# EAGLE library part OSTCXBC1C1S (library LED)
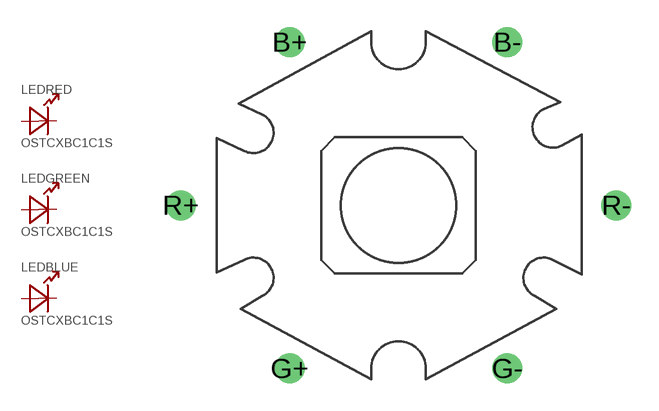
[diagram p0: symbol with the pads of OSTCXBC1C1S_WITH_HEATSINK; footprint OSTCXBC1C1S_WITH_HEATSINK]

Designator prefix LED; gates RED=LED GREEN=LED BLUE=LED

## OSTCXBC1C1S  [OSTCXBC1C1S_WITH_HEATSINK]
B+  BLUE:A  pas
B-  BLUE:C  pas
G+  GREEN:A  pas
G-  GREEN:C  pas
R+  RED:A  pas
R-  RED:C  pas

## Footprint OSTCXBC1C1S_WITH_HEATSINK (pad centres in mm)
OSTCXBC1C1S is a 3[W] 3 color LED. Red, Green, Blue. バランスがおかしい。 -- follow data is from Akituki -------------------------------- http://akizukidenshi.com/catalog/g/gI-03745/ Datasheet
drill 1.1: B+ -6,9; B- 6,9; G+ -6,-9; G- 6,-9; R+ -12,0; R- 12,0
